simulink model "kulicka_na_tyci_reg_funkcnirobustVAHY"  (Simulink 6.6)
settings: Solver=ode45  StartTime=0.0  StopTime=inf  FixedStep=0.01  RelTol=1e-3
undefined symbols (not defined in the file or in its folder): Humusoft, KA, KB, KC, KD, MF624, to, V
libraries: rtlib x4, simulink x1

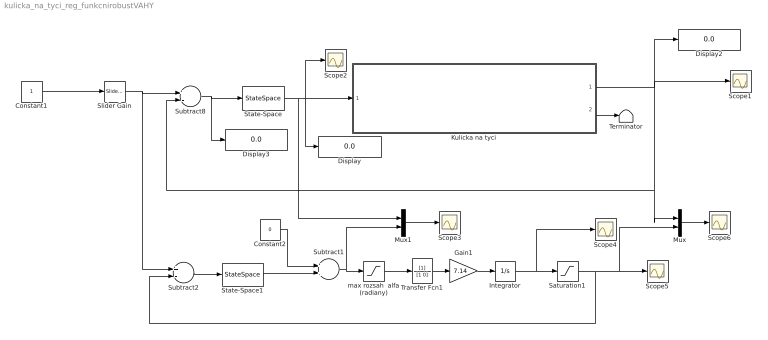
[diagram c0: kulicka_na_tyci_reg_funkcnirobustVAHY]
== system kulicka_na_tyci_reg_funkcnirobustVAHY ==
  Constant1 : Constant
  Constant2 : Constant  Value=0
  Display : Display
  Display2 : Display
  Display3 : Display
  Gain1 : Gain  Gain=7.14
  Integrator : Integrator
  Kulicka na tyci : Subsystem  TreatAsAtomicUnit=on  mask{Ts=0.02, IN_K=1, IN_R=2, OUT_S=1}
      mask prompts: Ts "Vzorkovaci perioda [s]"; IN_K "Cislo analog. vstupu - poloha kulicky"; IN_R "Cislo analog. vstupu - poloha ramane"; OUT_S "Cislo analog vystutpu - rizeni naklonu"
  Mux : Mux  Inputs=2
  Mux1 : Mux  Inputs=2
  Saturation1 : Saturate  UpperLimit=0.95  LowerLimit=0
  Scope{1..6} (6 alike) : Scope
  Slider Gain : simulink/Math Operations/Slider Gain  SystemSampleTime=-1  low=0  gain=0.5  high=1
  State-Space : StateSpace  A=KA  B=KB  C=KC  D=KD
  State-Space1 : StateSpace  A=KA  B=KB  C=KC  D=KD
  Subtract1 : Sum  OutScaling=2^-10
  Subtract2 : Sum  Inputs=+-  OutScaling=2^-10
  Subtract8 : Sum  Inputs=+-  OutScaling=2^-10
  Terminator : Terminator
  Transfer Fcn1 : TransferFcn  Denominator=[1 0]
  max rozsah  alfa (radiany) : Saturate  UpperLimit=0.01  LowerLimit=-0.01
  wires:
  Kulicka na tyci/1(kulicka) -> Scope1/1, Display2/1, Subtract8/2, Mux/1
  State-Space/1 -> Display/1, Kulicka na tyci/1(rameno), Scope2/1, Mux1/1
  Constant1/1 -> Slider Gain/1
  Transfer Fcn1/1 -> Gain1/1
  Integrator/1 -> Saturation1/1, Scope4/1
  Gain1/1 -> Integrator/1
  max rozsah  alfa (radiany)/1 -> Transfer Fcn1/1
  Saturation1/1 -> Subtract2/2, Scope5/1, Mux/2
  Subtract1/1 -> max rozsah  alfa (radiany)/1, Mux1/2
  Constant2/1 -> Subtract1/1
  Slider Gain/1 -> Subtract8/1, Subtract2/1
  Subtract8/1 -> State-Space/1, Display3/1
  State-Space1/1 -> Subtract1/2
  Subtract2/1 -> State-Space1/1
  Mux/1 -> Scope6/1
  Kulicka na tyci/2(rameno out) -> Terminator/1
  Mux1/1 -> Scope3/1

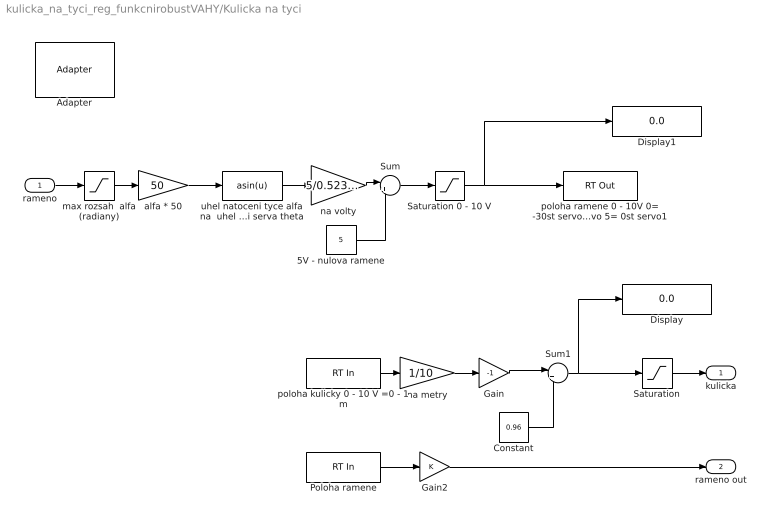
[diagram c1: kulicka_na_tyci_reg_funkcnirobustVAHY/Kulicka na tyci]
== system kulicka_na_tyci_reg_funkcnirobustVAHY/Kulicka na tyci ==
  rameno : Inport
  5V - nulova ramene : Constant  Value=5
  Adapter : rtlib/Adapter  SystemSampleTime=-1  DriverName=Humusoft/MF624  DriverAddress=4294967295  DriverOptions=0
  Constant : Constant  Value=0.96  SampleTime=-1
  Display : Display
  Display1 : Display
  Gain : Gain  Gain=-1
  Gain2 : Gain
  Poloha ramene : rtlib/RT In  SampleTime=Ts  Adapter=Adapter  IOClass=Analog Input  Channels=IN_R  SLDataType=double  MaxMissedTicks=inf  ShowMissedTicks=off  YieldWhenWaiting=on  AIORange=-10 to 10 V  AIOUnits=Volts  DIOMode=Bit  CIReset=never  CIEdge=rising  CIGate=none  EIQuadrature=quadruple  EIIndexPulse=reset  EIFilterFrequency=Inf  OIOParameters=[]
  Saturation : Saturate  UpperLimit=0.95  LowerLimit=0
  Saturation 0 - 10 V : Saturate  UpperLimit=10  LowerLimit=0
  Sum : Sum  Inputs=|++
  Sum1 : Sum  Inputs=|++
  alfa * 50 : Gain  Gain=50
  max rozsah  alfa (radiany) : Saturate  UpperLimit=0.01  LowerLimit=-0.01
  na metry : Gain  Gain=1/10
  na volty : Gain  Gain=5/0.52359877559830
  poloha kulicky 0 - 10 V =0 - 1 m : rtlib/RT In  SampleTime=Ts  Adapter=Adapter  IOClass=Analog Input  Channels=IN_K  SLDataType=double  MaxMissedTicks=inf  ShowMissedTicks=off  YieldWhenWaiting=on  AIORange=-10 to 10 V  AIOUnits=Volts  DIOMode=Bit  CIReset=never  CIEdge=rising  CIGate=none  EIQuadrature=quadruple  EIIndexPulse=reset  EIFilterFrequency=Inf  OIOParameters=[]
  poloha ramene 0 - 10V 0= -30st servo 10= +30st servo 5= 0st servo1 : rtlib/RT Out  SampleTime=Ts  Adapter=Adapter  IOClass=Analog Output  Channels=OUT_S  InitialValue=[0]  FinalValue=[0]  MaxMissedTicks=inf  ShowMissedTicks=off  YieldWhenWaiting=on  AIORange=-10 to 10 V  AIOUnits=Volts  DIOMode=Bit  OIOParameters=[]
  uhel natoceni tyce alfa na  uhel natoceni serva theta : Fcn  Expr=asin(u)
  kulicka : Outport
  rameno out : Outport  Port=2
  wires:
  poloha kulicky 0 - 10 V =0 - 1 m/1 -> na metry/1
  rameno/1 -> max rozsah  alfa (radiany)/1
  Saturation 0 - 10 V/1 -> Display1/1, poloha ramene 0 - 10V 0= -30st servo 10= +30st servo 5= 0st servo1/1
  Poloha ramene/1 -> Gain2/1
  Gain2/1 -> rameno out/1
  uhel natoceni tyce alfa na  uhel natoceni serva theta/1 -> na volty/1
  alfa * 50/1 -> uhel natoceni tyce alfa na  uhel natoceni serva theta/1
  max rozsah  alfa (radiany)/1 -> alfa * 50/1
  na volty/1 -> Sum/1
  5V - nulova ramene/1 -> Sum/2
  Sum/1 -> Saturation 0 - 10 V/1
  na metry/1 -> Gain/1
  Saturation/1 -> kulicka/1
  Gain/1 -> Sum1/1
  Sum1/1 -> Saturation/1, Display/1
  Constant/1 -> Sum1/2
